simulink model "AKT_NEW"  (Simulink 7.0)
settings: Solver=ode45  StartTime=0.0  StopTime=10  RelTol=1e-3

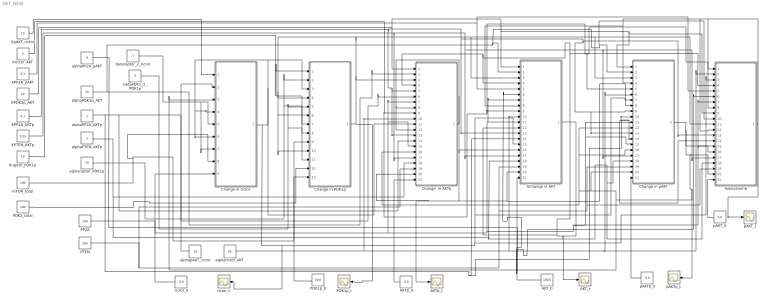
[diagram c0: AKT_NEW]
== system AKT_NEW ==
  AKT_0 : Constant  Orientation=left  Value=100.0  OutDataType=sfix(16)  OutScaling=2^0
  AKT_t : Scope
  AKTp_0 : Constant  Orientation=left  Value=0.0  OutDataType=sfix(16)  OutScaling=2^0
  AKTp_t : Scope
  Change  in AKTp : Subsystem
  Change in PDK1p : Subsystem
  Change in pAKT : Subsystem
  Change in rictor : Subsystem
  KPDK1p_AKT : Constant  Value=10  OutDataType=sfix(16)  OutScaling=2^0
  KPP2A_AKTp : Constant  Value=0.1  OutDataType=sfix(16)  OutScaling=2^0
  KPP2A_pAKT : Constant  Value=0.1  OutDataType=sfix(16)  OutScaling=2^0
  KPTEN_AKTp : Constant  Value=0.25  OutDataType=sfix(16)  OutScaling=2^0
  KpAKT_rictor : Constant  Value=10  OutDataType=sfix(16)  OutScaling=2^0
  Kraptor_PDK1p : Constant  Value=10  OutDataType=sfix(16)  OutScaling=2^0
  Krictor_AKT : Constant  Value=5  OutDataType=sfix(16)  OutScaling=2^0
  PDK1_total : Constant  Value=100  OutDataType=sfix(16)  OutScaling=2^0
  PDK1p_0 : Constant  Orientation=left  Value=50.0  OutDataType=sfix(16)  OutScaling=2^0
  PDK1p_t : Scope
  PP2A : Constant  Value=150  OutDataType=sfix(16)  OutScaling=2^0
  PTEN : Constant  Value=200  OutDataType=sfix(16)  OutScaling=2^0
  SChange in AKT : Subsystem
  Subsystem6 : Subsystem
  alphaPDK1p_AKT : Constant  Value=20  OutDataType=sfix(16)  OutScaling=2^0
  alphaPP2A_AKTp : Constant  OutDataType=sfix(16)  OutScaling=2^0
  alphaPP2A_pAKT : Constant  Value=4  OutDataType=sfix(16)  OutScaling=2^0
  alphaPTEN_AKTp : Constant  OutDataType=sfix(16)  OutScaling=2^0
  alphapAKT_rictor : Constant  Orientation=left  Value=10  OutDataType=sfix(16)  OutScaling=2^0
  alpharaptor_PDK1p : Constant  Value=10  OutDataType=sfix(16)  OutScaling=2^0
  alpharictor_AKT : Constant  Value=20  OutDataType=sfix(16)  OutScaling=2^0
  betaPDK1_2_PDK1p : Constant  Value=5  OutDataType=sfix(16)  OutScaling=2^0
  betaraptor_2_rictor : Constant  OutDataType=sfix(16)  OutScaling=2^0
  mTOR_total : Constant  Value=100  OutDataType=sfix(16)  OutScaling=2^0
  pAKT_0 : Constant  Orientation=left  Value=0.0  OutDataType=sfix(16)  OutScaling=2^0
  pAKT_t : Scope
  pAKTp_0 : Constant  Orientation=left  Value=0.0  OutDataType=sfix(16)  OutScaling=2^0
  pAKTp_t : Scope
  rictor_0 : Constant  Orientation=left  Value=0.0  OutDataType=sfix(16)  OutScaling=2^0
  rictor_t : Scope
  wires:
  Change in pAKT/1(Out1) -> Subsystem6/20(In21), Change  in AKTp/16(In16), Change in pAKT/16(In16), Change in pAKT/12(In12), Change in pAKT/20(In21), Change in rictor/3(In3), pAKTp_t/1, Subsystem6/16(In16)
  KpAKT_rictor/1 -> Change in rictor/1(In1)
  Krictor_AKT/1 -> SChange in AKT/9(In9), Subsystem6/1(In1), Change in pAKT/5(In5), Change  in AKTp/9(In9)
  KPDK1p_AKT/1 -> SChange in AKT/1(In1), Subsystem6/9(In9), Change in pAKT/1(In1), Change  in AKTp/1(In1)
  KPTEN_AKTp/1 -> Change  in AKTp/17(In17), SChange in AKT/17(In17), Change in pAKT/17(In17), Subsystem6/17(In17)
  Kraptor_PDK1p/1 -> Change in PDK1p/1(In1), Change in PDK1p/7(In9)
  alphapAKT_rictor/1 -> Change in rictor/2(In2)
  alphaPP2A_pAKT/1 -> SChange in AKT/6(In6), Subsystem6/6(In6)
  alphaPDK1p_AKT/1 -> Change  in AKTp/2(In2), SChange in AKT/2(In2), Subsystem6/10(In10), Change in pAKT/2(In2)
  alphaPTEN_AKTp/1 -> Change  in AKTp/18(In18), SChange in AKT/18(In18), Change in pAKT/18(In18), Subsystem6/18(In18)
  alpharaptor_PDK1p/1 -> Change in PDK1p/2(In2), Change in PDK1p/8(In10)
  PP2A/1 -> Change in pAKT/11(In11), Change in pAKT/15(In15), Subsystem6/7(In7), Subsystem6/15(In15), SChange in AKT/7(In7), SChange in AKT/15(In15), Change  in AKTp/7(In7), Change  in AKTp/15(In15)
  PTEN/1 -> Change  in AKTp/19(In19), SChange in AKT/19(In19), Change in pAKT/19(In19), Subsystem6/19(In19)
  betaPDK1_2_PDK1p/1 -> Change in PDK1p/5(In5), Change in PDK1p/11(In13)
  mTOR_total/1 -> Change in rictor/8(In10), Change in PDK1p/9(In11)
  PDK1_total/1 -> Change in PDK1p/12(In14)
  Change in rictor/1(Out1) -> Change  in AKTp/11(In11), Change in PDK1p/3(In3), Change in rictor/4(In4), Change in rictor/6(In6), SChange in AKT/11(In11), Change in pAKT/7(In7), Subsystem6/3(In3), rictor_t/1
  alphaPP2A_AKTp/1 -> Change  in AKTp/6(In6), Change  in AKTp/14(In14), SChange in AKT/14(In14), Change in pAKT/14(In14), Subsystem6/14(In14), Change in pAKT/10(In10)
  Change  in AKTp/1(Out1) -> Change  in AKTp/12(In12), Change  in AKTp/8(In8), Change  in AKTp/20(In21), AKTp_t/1, Change in pAKT/8(In8), SChange in AKT/20(In21), SChange in AKT/16(In16)
  Subsystem6/1(Out1) -> Subsystem6/12(In12), Change in pAKT/4(In4), SChange in AKT/8(In8), Subsystem6/8(In8), pAKT_t/1
  SChange in AKT/1(Out1) -> Subsystem6/4(In4), SChange in AKT/4(In4), Change  in AKTp/4(In4), SChange in AKT/12(In12), AKT_t/1
  rictor_0/1 -> Change in rictor/9(In7)
  PDK1p_0/1 -> Change in PDK1p/13(In7)
  AKTp_0/1 -> Change  in AKTp/21(In20)
  AKT_0/1 -> SChange in AKT/21(In20)
  pAKTp_0/1 -> Change in pAKT/21(In20)
  pAKT_0/1 -> Subsystem6/21(In20)
  betaraptor_2_rictor/1 -> Change in rictor/5(In5), Change in rictor/7(In9)
  KPP2A_pAKT/1 -> Subsystem6/5(In5), SChange in AKT/5(In5)
  KPP2A_AKTp/1 -> Change  in AKTp/5(In5), Change  in AKTp/13(In13), Change in pAKT/9(In9), Change in pAKT/13(In13), Subsystem6/13(In13), SChange in AKT/13(In13)
  alpharictor_AKT/1 -> Change  in AKTp/10(In10), SChange in AKT/10(In10), Change in pAKT/6(In6), Subsystem6/2(In2)
  Change in PDK1p/1(Out1) -> Change  in AKTp/3(In3), Change in PDK1p/4(In4), Change in PDK1p/10(In12), Change in PDK1p/6(In6), SChange in AKT/3(In3), Change in pAKT/3(In3), Subsystem6/11(In11), PDK1p_t/1

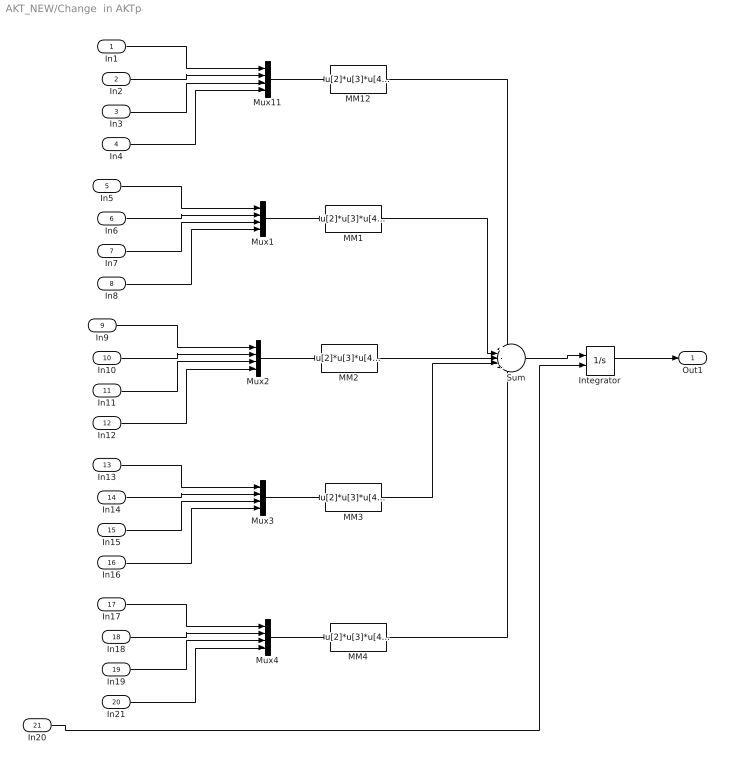
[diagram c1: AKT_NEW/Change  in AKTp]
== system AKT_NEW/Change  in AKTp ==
  In1 : Inport  OutDataType=sfix(16)  OutScaling=2^0
  In2 : Inport  Port=2  OutDataType=sfix(16)  OutScaling=2^0
  In3 : Inport  Port=3  OutDataType=sfix(16)  OutScaling=2^0
  In4 : Inport  Port=4  OutDataType=sfix(16)  OutScaling=2^0
  In5 : Inport  Port=5  OutDataType=sfix(16)  OutScaling=2^0
  In6 : Inport  Port=6  OutDataType=sfix(16)  OutScaling=2^0
  In7 : Inport  Port=7  OutDataType=sfix(16)  OutScaling=2^0
  In8 : Inport  Port=8  OutDataType=sfix(16)  OutScaling=2^0
  In9 : Inport  Port=9  OutDataType=sfix(16)  OutScaling=2^0
  In10 : Inport  Port=10  OutDataType=sfix(16)  OutScaling=2^0
  In11 : Inport  Port=11  OutDataType=sfix(16)  OutScaling=2^0
  In12 : Inport  Port=12  OutDataType=sfix(16)  OutScaling=2^0
  In13 : Inport  Port=13  OutDataType=sfix(16)  OutScaling=2^0
  In14 : Inport  Port=14  OutDataType=sfix(16)  OutScaling=2^0
  In15 : Inport  Port=15  OutDataType=sfix(16)  OutScaling=2^0
  In16 : Inport  Port=16  OutDataType=sfix(16)  OutScaling=2^0
  In17 : Inport  Port=17  OutDataType=sfix(16)  OutScaling=2^0
  In18 : Inport  Port=18  OutDataType=sfix(16)  OutScaling=2^0
  In19 : Inport  Port=19  OutDataType=sfix(16)  OutScaling=2^0
  In21 : Inport  Port=20  OutDataType=sfix(16)  OutScaling=2^0
  In20 : Inport  Port=21  OutDataType=sfix(16)  OutScaling=2^0
  Integrator : Integrator  InitialConditionSource=external
  MM{1..4,12} (5 alike) : Fcn  Expr=u[2]*u[3]*u[4]/(u[1]+u[4])
  Mux{1..4,11} (5 alike) : Mux
  Sum : Sum  Inputs=+--+-  OutDataType=sfix(16)  OutScaling=2^0
  Out1 : Outport  OutDataType=sfix(16)  OutScaling=2^0
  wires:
  Mux11/1 -> MM12/1
  In1/1 -> Mux11/1
  In2/1 -> Mux11/2
  In3/1 -> Mux11/3
  In4/1 -> Mux11/4
  Mux1/1 -> MM1/1
  In5/1 -> Mux1/1
  In6/1 -> Mux1/2
  In7/1 -> Mux1/3
  In8/1 -> Mux1/4
  Mux2/1 -> MM2/1
  In9/1 -> Mux2/1
  In10/1 -> Mux2/2
  In11/1 -> Mux2/3
  In12/1 -> Mux2/4
  Mux3/1 -> MM3/1
  In13/1 -> Mux3/1
  In14/1 -> Mux3/2
  In15/1 -> Mux3/3
  In16/1 -> Mux3/4
  Mux4/1 -> MM4/1
  In17/1 -> Mux4/1
  In18/1 -> Mux4/2
  In19/1 -> Mux4/3
  In21/1 -> Mux4/4
  MM12/1 -> Sum/1
  MM1/1 -> Sum/2
  MM2/1 -> Sum/3
  MM3/1 -> Sum/4
  MM4/1 -> Sum/5
  Sum/1 -> Integrator/1
  Integrator/1 -> Out1/1
  In20/1 -> Integrator/2

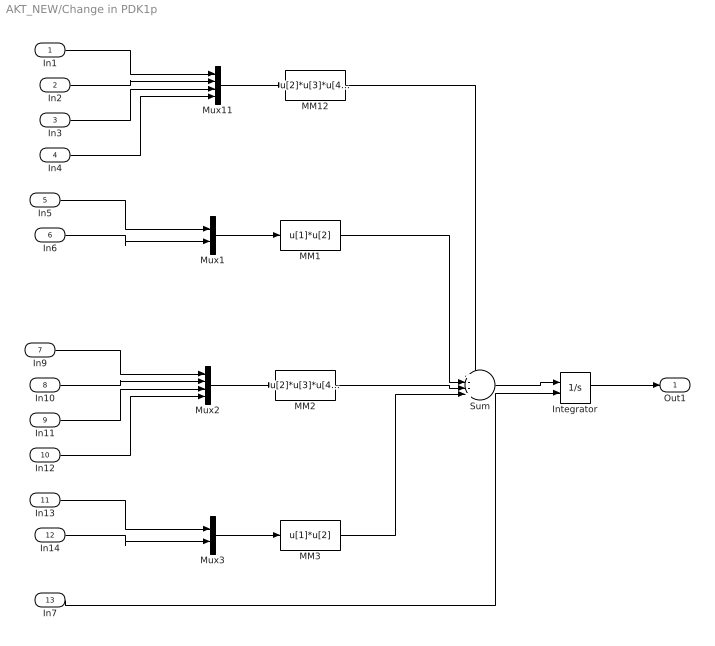
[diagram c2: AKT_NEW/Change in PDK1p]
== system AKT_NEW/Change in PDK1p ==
  In1 : Inport  OutDataType=sfix(16)  OutScaling=2^0
  In2 : Inport  Port=2  OutDataType=sfix(16)  OutScaling=2^0
  In3 : Inport  Port=3  OutDataType=sfix(16)  OutScaling=2^0
  In4 : Inport  Port=4  OutDataType=sfix(16)  OutScaling=2^0
  In5 : Inport  Port=5  OutDataType=sfix(16)  OutScaling=2^0
  In6 : Inport  Port=6  OutDataType=sfix(16)  OutScaling=2^0
  In9 : Inport  Port=7  OutDataType=sfix(16)  OutScaling=2^0
  In10 : Inport  Port=8  OutDataType=sfix(16)  OutScaling=2^0
  In11 : Inport  Port=9  OutDataType=sfix(16)  OutScaling=2^0
  In12 : Inport  Port=10  OutDataType=sfix(16)  OutScaling=2^0
  In13 : Inport  Port=11  OutDataType=sfix(16)  OutScaling=2^0
  In14 : Inport  Port=12  OutDataType=sfix(16)  OutScaling=2^0
  In7 : Inport  Port=13  OutDataType=sfix(16)  OutScaling=2^0
  Integrator : Integrator  InitialConditionSource=external  InitialCondition=50
  MM1 : Fcn  Expr=u[1]*u[2]
  MM12 : Fcn  Expr=u[2]*u[3]*u[4]/(u[1]+u[4])
  MM2 : Fcn  Expr=u[2]*u[3]*u[4]/(u[1]+u[4])
  MM3 : Fcn  Expr=u[1]*u[2]
  Mux1 : Mux  Inputs=2
  Mux11 : Mux
  Mux2 : Mux
  Mux3 : Mux  Inputs=2
  Sum : Sum  Inputs=+--+  OutDataType=sfix(16)  OutScaling=2^0
  Out1 : Outport  OutDataType=sfix(16)  OutScaling=2^0
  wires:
  Mux11/1 -> MM12/1
  In1/1 -> Mux11/1
  In2/1 -> Mux11/2
  In3/1 -> Mux11/3
  In4/1 -> Mux11/4
  Mux1/1 -> MM1/1
  In5/1 -> Mux1/1
  In6/1 -> Mux1/2
  Mux2/1 -> MM2/1
  In9/1 -> Mux2/1
  In10/1 -> Mux2/2
  In11/1 -> Mux2/3
  In12/1 -> Mux2/4
  Mux3/1 -> MM3/1
  In13/1 -> Mux3/1
  In14/1 -> Mux3/2
  MM12/1 -> Sum/1
  MM1/1 -> Sum/2
  MM2/1 -> Sum/3
  MM3/1 -> Sum/4
  Sum/1 -> Integrator/1
  Integrator/1 -> Out1/1
  In7/1 -> Integrator/2

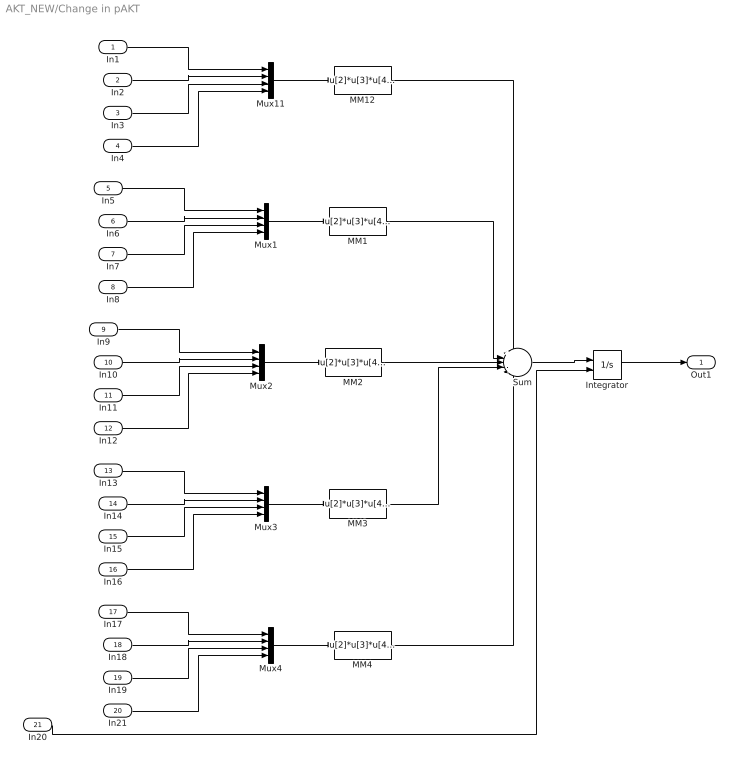
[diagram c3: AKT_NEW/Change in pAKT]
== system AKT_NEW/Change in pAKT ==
  In1 : Inport  OutDataType=sfix(16)  OutScaling=2^0
  In2 : Inport  Port=2  OutDataType=sfix(16)  OutScaling=2^0
  In3 : Inport  Port=3  OutDataType=sfix(16)  OutScaling=2^0
  In4 : Inport  Port=4  OutDataType=sfix(16)  OutScaling=2^0
  In5 : Inport  Port=5  OutDataType=sfix(16)  OutScaling=2^0
  In6 : Inport  Port=6  OutDataType=sfix(16)  OutScaling=2^0
  In7 : Inport  Port=7  OutDataType=sfix(16)  OutScaling=2^0
  In8 : Inport  Port=8  OutDataType=sfix(16)  OutScaling=2^0
  In9 : Inport  Port=9  OutDataType=sfix(16)  OutScaling=2^0
  In10 : Inport  Port=10  OutDataType=sfix(16)  OutScaling=2^0
  In11 : Inport  Port=11  OutDataType=sfix(16)  OutScaling=2^0
  In12 : Inport  Port=12  OutDataType=sfix(16)  OutScaling=2^0
  In13 : Inport  Port=13  OutDataType=sfix(16)  OutScaling=2^0
  In14 : Inport  Port=14  OutDataType=sfix(16)  OutScaling=2^0
  In15 : Inport  Port=15  OutDataType=sfix(16)  OutScaling=2^0
  In16 : Inport  Port=16  OutDataType=sfix(16)  OutScaling=2^0
  In17 : Inport  Port=17  OutDataType=sfix(16)  OutScaling=2^0
  In18 : Inport  Port=18  OutDataType=sfix(16)  OutScaling=2^0
  In19 : Inport  Port=19  OutDataType=sfix(16)  OutScaling=2^0
  In21 : Inport  Port=20  OutDataType=sfix(16)  OutScaling=2^0
  In20 : Inport  Port=21  OutDataType=sfix(16)  OutScaling=2^0
  Integrator : Integrator  InitialConditionSource=external
  MM{1..4,12} (5 alike) : Fcn  Expr=u[2]*u[3]*u[4]/(u[1]+u[4])
  Mux{1..4,11} (5 alike) : Mux
  Sum : Sum  Inputs=++---  OutDataType=sfix(16)  OutScaling=2^0
  Out1 : Outport  OutDataType=sfix(16)  OutScaling=2^0
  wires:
  Mux11/1 -> MM12/1
  In1/1 -> Mux11/1
  In2/1 -> Mux11/2
  In3/1 -> Mux11/3
  In4/1 -> Mux11/4
  Mux1/1 -> MM1/1
  In5/1 -> Mux1/1
  In6/1 -> Mux1/2
  In7/1 -> Mux1/3
  In8/1 -> Mux1/4
  Mux2/1 -> MM2/1
  In9/1 -> Mux2/1
  In10/1 -> Mux2/2
  In11/1 -> Mux2/3
  In12/1 -> Mux2/4
  Mux3/1 -> MM3/1
  In13/1 -> Mux3/1
  In14/1 -> Mux3/2
  In15/1 -> Mux3/3
  In16/1 -> Mux3/4
  Mux4/1 -> MM4/1
  In17/1 -> Mux4/1
  In18/1 -> Mux4/2
  In19/1 -> Mux4/3
  In21/1 -> Mux4/4
  MM12/1 -> Sum/1
  MM1/1 -> Sum/2
  MM2/1 -> Sum/3
  MM3/1 -> Sum/4
  MM4/1 -> Sum/5
  Sum/1 -> Integrator/1
  Integrator/1 -> Out1/1
  In20/1 -> Integrator/2

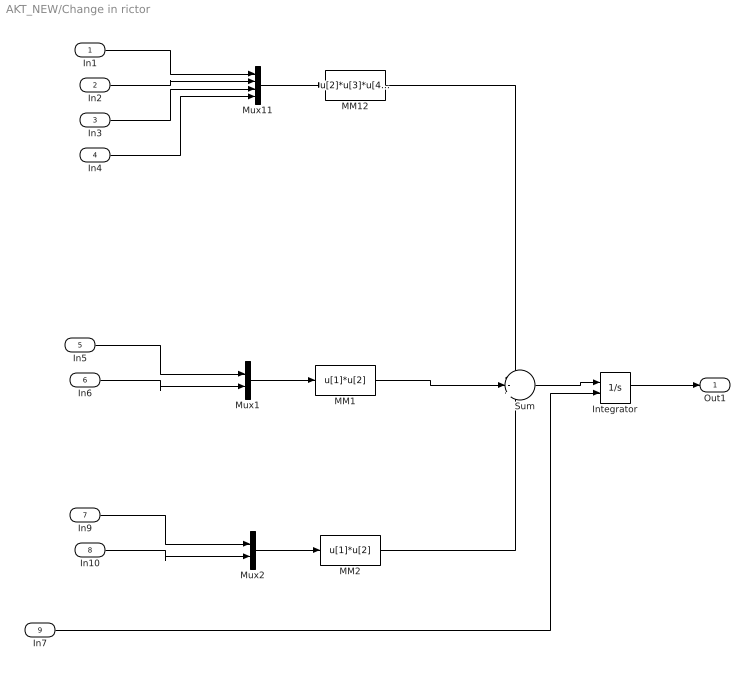
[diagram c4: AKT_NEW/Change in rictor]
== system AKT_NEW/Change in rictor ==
  In1 : Inport  OutDataType=sfix(16)  OutScaling=2^0
  In2 : Inport  Port=2  OutDataType=sfix(16)  OutScaling=2^0
  In3 : Inport  Port=3  OutDataType=sfix(16)  OutScaling=2^0
  In4 : Inport  Port=4  OutDataType=sfix(16)  OutScaling=2^0
  In5 : Inport  Port=5  OutDataType=sfix(16)  OutScaling=2^0
  In6 : Inport  Port=6  OutDataType=sfix(16)  OutScaling=2^0
  In9 : Inport  Port=7  OutDataType=sfix(16)  OutScaling=2^0
  In10 : Inport  Port=8  OutDataType=sfix(16)  OutScaling=2^0
  In7 : Inport  Port=9  OutDataType=sfix(16)  OutScaling=2^0
  Integrator : Integrator  InitialConditionSource=external
  MM1 : Fcn  Expr=u[1]*u[2]
  MM12 : Fcn  Expr=u[2]*u[3]*u[4]/(u[1]+u[4])
  MM2 : Fcn  Expr=u[1]*u[2]
  Mux1 : Mux  Inputs=2
  Mux11 : Mux
  Mux2 : Mux  Inputs=2
  Sum : Sum  Inputs=--+  OutDataType=sfix(16)  OutScaling=2^0
  Out1 : Outport  OutDataType=sfix(16)  OutScaling=2^0
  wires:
  Mux11/1 -> MM12/1
  In1/1 -> Mux11/1
  In2/1 -> Mux11/2
  In3/1 -> Mux11/3
  In4/1 -> Mux11/4
  Mux1/1 -> MM1/1
  In5/1 -> Mux1/1
  In6/1 -> Mux1/2
  Mux2/1 -> MM2/1
  In9/1 -> Mux2/1
  In10/1 -> Mux2/2
  MM12/1 -> Sum/1
  Sum/1 -> Integrator/1
  Integrator/1 -> Out1/1
  MM1/1 -> Sum/2
  MM2/1 -> Sum/3
  In7/1 -> Integrator/2

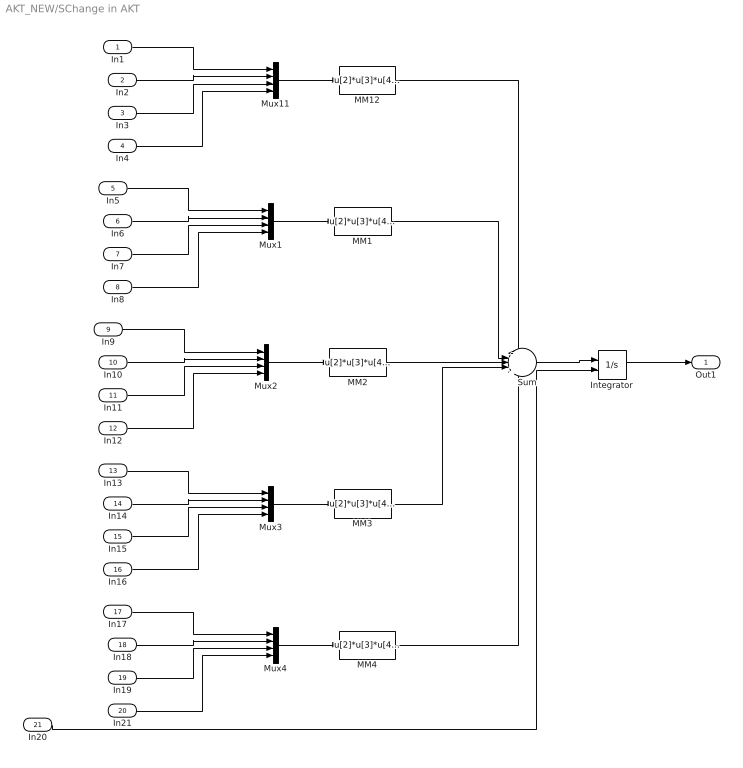
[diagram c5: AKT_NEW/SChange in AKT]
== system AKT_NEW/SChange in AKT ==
  In1 : Inport  OutDataType=sfix(16)  OutScaling=2^0
  In2 : Inport  Port=2  OutDataType=sfix(16)  OutScaling=2^0
  In3 : Inport  Port=3  OutDataType=sfix(16)  OutScaling=2^0
  In4 : Inport  Port=4  OutDataType=sfix(16)  OutScaling=2^0
  In5 : Inport  Port=5  OutDataType=sfix(16)  OutScaling=2^0
  In6 : Inport  Port=6  OutDataType=sfix(16)  OutScaling=2^0
  In7 : Inport  Port=7  OutDataType=sfix(16)  OutScaling=2^0
  In8 : Inport  Port=8  OutDataType=sfix(16)  OutScaling=2^0
  In9 : Inport  Port=9  OutDataType=sfix(16)  OutScaling=2^0
  In10 : Inport  Port=10  OutDataType=sfix(16)  OutScaling=2^0
  In11 : Inport  Port=11  OutDataType=sfix(16)  OutScaling=2^0
  In12 : Inport  Port=12  OutDataType=sfix(16)  OutScaling=2^0
  In13 : Inport  Port=13  OutDataType=sfix(16)  OutScaling=2^0
  In14 : Inport  Port=14  OutDataType=sfix(16)  OutScaling=2^0
  In15 : Inport  Port=15  OutDataType=sfix(16)  OutScaling=2^0
  In16 : Inport  Port=16  OutDataType=sfix(16)  OutScaling=2^0
  In17 : Inport  Port=17  OutDataType=sfix(16)  OutScaling=2^0
  In18 : Inport  Port=18  OutDataType=sfix(16)  OutScaling=2^0
  In19 : Inport  Port=19  OutDataType=sfix(16)  OutScaling=2^0
  In21 : Inport  Port=20  OutDataType=sfix(16)  OutScaling=2^0
  In20 : Inport  Port=21  OutDataType=sfix(16)  OutScaling=2^0
  Integrator : Integrator  InitialConditionSource=external  InitialCondition=100
  MM{1..4,12} (5 alike) : Fcn  Expr=u[2]*u[3]*u[4]/(u[1]+u[4])
  Mux{1..4,11} (5 alike) : Mux
  Sum : Sum  Inputs=-+-++  OutDataType=sfix(16)  OutScaling=2^0
  Out1 : Outport  OutDataType=sfix(16)  OutScaling=2^0
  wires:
  Mux11/1 -> MM12/1
  In1/1 -> Mux11/1
  In2/1 -> Mux11/2
  In3/1 -> Mux11/3
  In4/1 -> Mux11/4
  Mux1/1 -> MM1/1
  In5/1 -> Mux1/1
  In6/1 -> Mux1/2
  In7/1 -> Mux1/3
  In8/1 -> Mux1/4
  Mux2/1 -> MM2/1
  In9/1 -> Mux2/1
  In10/1 -> Mux2/2
  In11/1 -> Mux2/3
  In12/1 -> Mux2/4
  Mux3/1 -> MM3/1
  In13/1 -> Mux3/1
  In14/1 -> Mux3/2
  In15/1 -> Mux3/3
  In16/1 -> Mux3/4
  Mux4/1 -> MM4/1
  In17/1 -> Mux4/1
  In18/1 -> Mux4/2
  In19/1 -> Mux4/3
  In21/1 -> Mux4/4
  MM12/1 -> Sum/1
  MM1/1 -> Sum/2
  MM2/1 -> Sum/3
  MM3/1 -> Sum/4
  MM4/1 -> Sum/5
  Sum/1 -> Integrator/1
  Integrator/1 -> Out1/1
  In20/1 -> Integrator/2

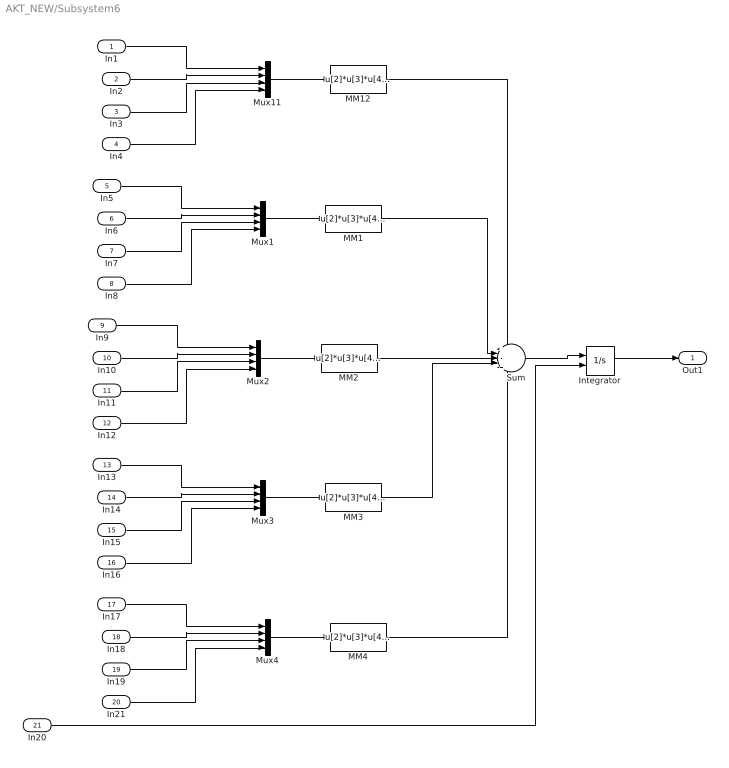
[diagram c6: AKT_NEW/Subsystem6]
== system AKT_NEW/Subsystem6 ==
  In1 : Inport  OutDataType=sfix(16)  OutScaling=2^0
  In2 : Inport  Port=2  OutDataType=sfix(16)  OutScaling=2^0
  In3 : Inport  Port=3  OutDataType=sfix(16)  OutScaling=2^0
  In4 : Inport  Port=4  OutDataType=sfix(16)  OutScaling=2^0
  In5 : Inport  Port=5  OutDataType=sfix(16)  OutScaling=2^0
  In6 : Inport  Port=6  OutDataType=sfix(16)  OutScaling=2^0
  In7 : Inport  Port=7  OutDataType=sfix(16)  OutScaling=2^0
  In8 : Inport  Port=8  OutDataType=sfix(16)  OutScaling=2^0
  In9 : Inport  Port=9  OutDataType=sfix(16)  OutScaling=2^0
  In10 : Inport  Port=10  OutDataType=sfix(16)  OutScaling=2^0
  In11 : Inport  Port=11  OutDataType=sfix(16)  OutScaling=2^0
  In12 : Inport  Port=12  OutDataType=sfix(16)  OutScaling=2^0
  In13 : Inport  Port=13  OutDataType=sfix(16)  OutScaling=2^0
  In14 : Inport  Port=14  OutDataType=sfix(16)  OutScaling=2^0
  In15 : Inport  Port=15  OutDataType=sfix(16)  OutScaling=2^0
  In16 : Inport  Port=16  OutDataType=sfix(16)  OutScaling=2^0
  In17 : Inport  Port=17  OutDataType=sfix(16)  OutScaling=2^0
  In18 : Inport  Port=18  OutDataType=sfix(16)  OutScaling=2^0
  In19 : Inport  Port=19  OutDataType=sfix(16)  OutScaling=2^0
  In21 : Inport  Port=20  OutDataType=sfix(16)  OutScaling=2^0
  In20 : Inport  Port=21  OutDataType=sfix(16)  OutScaling=2^0
  Integrator : Integrator  InitialConditionSource=external
  MM{1..4,12} (5 alike) : Fcn  Expr=u[2]*u[3]*u[4]/(u[1]+u[4])
  Mux{1..4,11} (5 alike) : Mux
  Sum : Sum  Inputs=+--++  OutDataType=sfix(16)  OutScaling=2^0
  Out1 : Outport  OutDataType=sfix(16)  OutScaling=2^0
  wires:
  Mux11/1 -> MM12/1
  In1/1 -> Mux11/1
  In2/1 -> Mux11/2
  In3/1 -> Mux11/3
  In4/1 -> Mux11/4
  Mux1/1 -> MM1/1
  In5/1 -> Mux1/1
  In6/1 -> Mux1/2
  In7/1 -> Mux1/3
  In8/1 -> Mux1/4
  Mux2/1 -> MM2/1
  In9/1 -> Mux2/1
  In10/1 -> Mux2/2
  In11/1 -> Mux2/3
  In12/1 -> Mux2/4
  Mux3/1 -> MM3/1
  In13/1 -> Mux3/1
  In14/1 -> Mux3/2
  In15/1 -> Mux3/3
  In16/1 -> Mux3/4
  Mux4/1 -> MM4/1
  In17/1 -> Mux4/1
  In18/1 -> Mux4/2
  In19/1 -> Mux4/3
  In21/1 -> Mux4/4
  MM12/1 -> Sum/1
  MM1/1 -> Sum/2
  MM2/1 -> Sum/3
  MM3/1 -> Sum/4
  MM4/1 -> Sum/5
  Sum/1 -> Integrator/1
  Integrator/1 -> Out1/1
  In20/1 -> Integrator/2
